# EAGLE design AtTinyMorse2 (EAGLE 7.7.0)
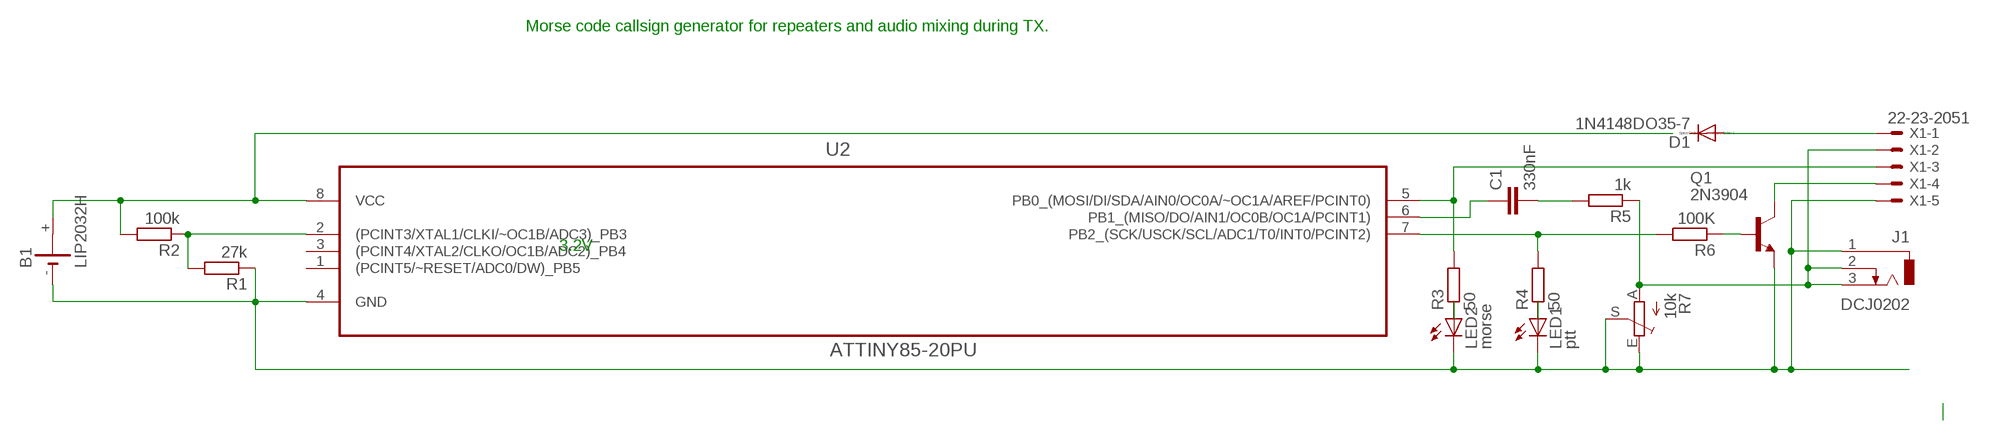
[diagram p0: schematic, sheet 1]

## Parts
B1  LIP2032H  CR2032H  [CR2032H]
C1  330nF  C5/2.5  [C5B2.5]
D1  1N4148DO35-7  [DO35-7]
J1  DCJ0202  [DCJ0202]
LED1  ptt  LED3MM  [LED3MM]
LED2  morse  LED3MM  [LED3MM]
Q1  2N3904  [TO92]
R1  27k  R-EU_0204/7  [0204/7]
R2  100k  R-EU_0204/7  [0204/7]
R3  50  R-EU_0204/7  [0204/7]
R4  50  R-EU_0204/7  [0204/7]
R5  1k  R-EU_0204/7  [0204/7]
R6  100K  R-EU_0204/7  [0204/7]
R7  10k  TRIM_EU-LI10  [LI10]
U2  ATTINY85-20PU  [DIP254P762X533-8]
X1  22-23-2051  [22-23-2051]

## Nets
N$1: LED2.A R3.1
N$2: LED1.A R4.1
N$4: Q1.1(C) X1.4
N$9: C1.2 R5.2
N$10: J1.2 J1.3 R5.1 R7.A X1.2
N$12: Q1.2(B) R6.1
N$13: D1.A X1.1
N$14: B1.- J1.1 LED1.K(C) LED2.K(C) R1.1 R7.E R7.S U2.4(GND) X1.5
N$15: B1.+ R2.2 U2.8(VCC)
N$16: R1.2 R2.1 U2.2((PCINT3/XTAL1/CLKI/~OC1B/ADC3)_PB3)
N$19: Q1.3(E)
N$20: R4.2 R6.2 U2.7(PB2_(SCK/USCK/SCL/ADC1/T0/INT0/PCINT2))
N$21: R3.2 U2.5(PB0_(MOSI/DI/SDA/AIN0/OC0A/~OC1A/AREF/PCINT0)) X1.3
N$22: C1.1 U2.6(PB1_(MISO/DO/AIN1/OC0B/OC1A/PCINT1))
Unconnected: B1.+@1(+) D1.C U2.1((PCINT5/~RESET/ADC0/DW)_PB5) U2.3((PCINT4/XTAL2/CLKO/OC1B/ADC2)_PB4)

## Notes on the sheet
- Morse code callsign generator for repeaters and audio mixing during TX.
- 3.2V

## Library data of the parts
B1 = battery:CR2032H: LI BATTERY Varta
C1 = capacitor-wima:C: CAPACITOR
D1 = diode:1N4148: DIODE
J1 = con-jack:DCJ0202: DC POWER JACK Source: DCJ0202.pdf; OC_FARNELL: unknown; OC_NEWARK: unknown
LED1 LED2 = led:LED: LED
Q1 = transistor-npn:2N3904: NPN Transistor
R1-R6 = resistor:R-EU_: RESISTOR, European symbol
R7 = pot:TRIM_EU-: POTENTIOMETER
U2 = Atmel_By_element14_Batch_1-00:ATTINY85-20PU: 8-bit Microcontroller with In-System Programmable Flash; MPN: ATTINY85-20PU; OC_FARNELL: 1455162; OC_NEWARK: 58M3796; PACKAGE: PDIP-8; SUPPLIER: Atmel
X1 = con-molex:22-23-2051: .100" (2.54mm) Center Header - 5 Pin; MF: MOLEX; MPN: 22-23-2051; OC_FARNELL: 1462952; OC_NEWARK: 38C9178

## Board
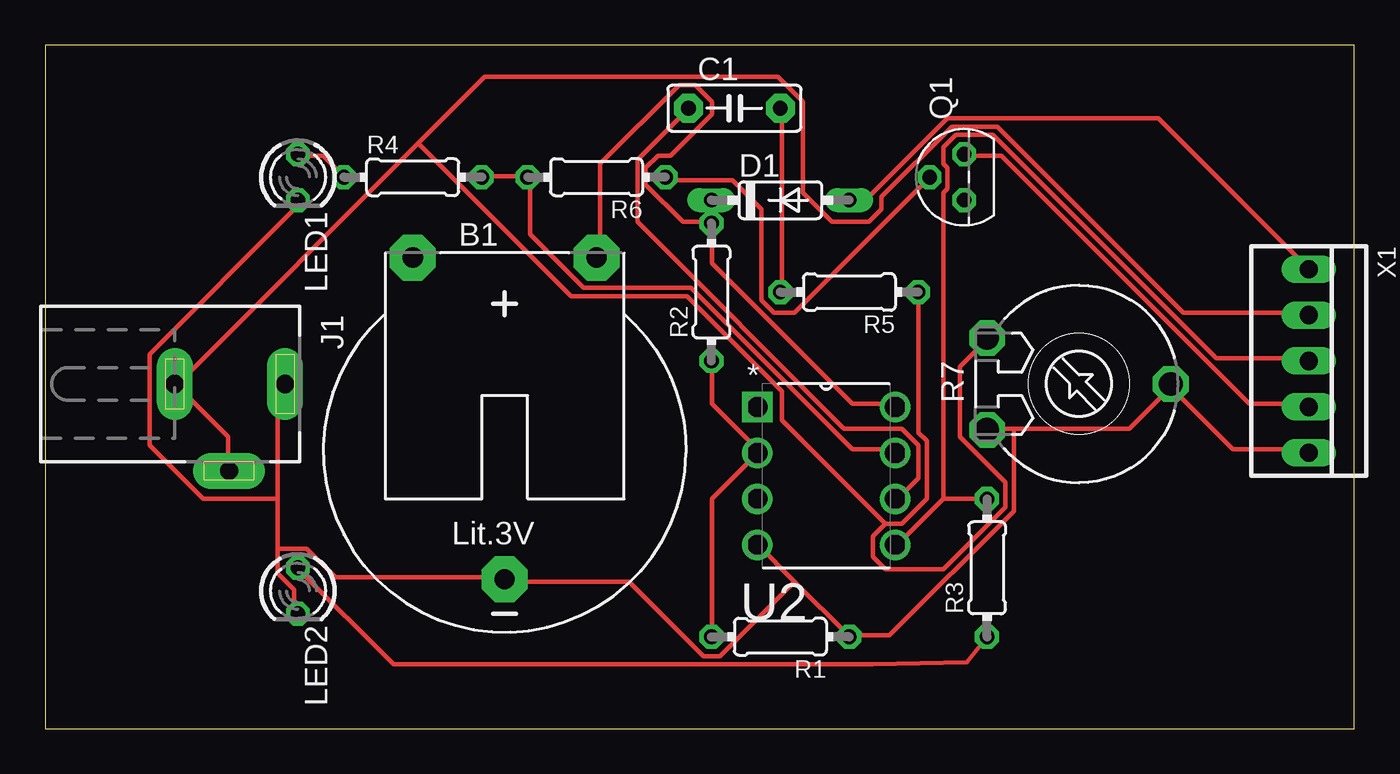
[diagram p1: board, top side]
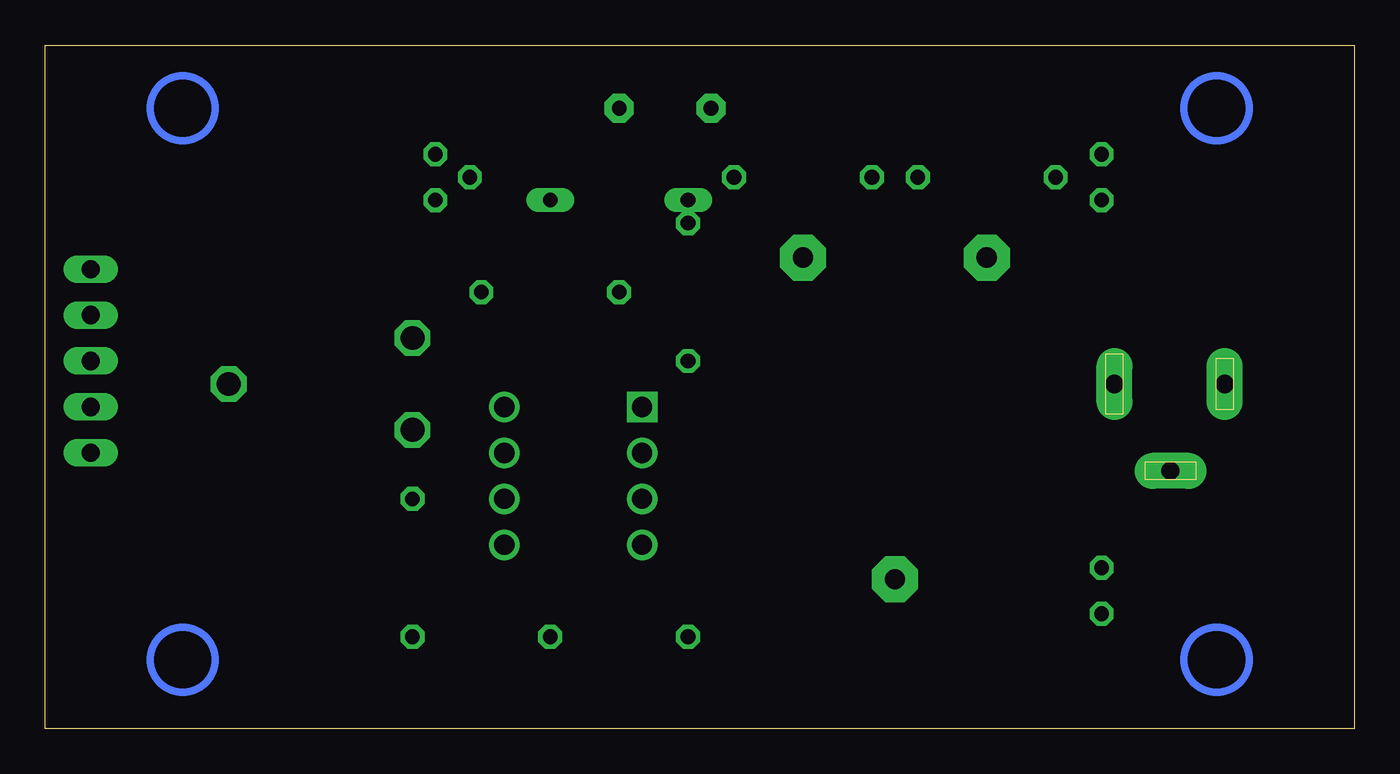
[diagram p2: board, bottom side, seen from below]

Size 72.37 x 37.77 mm. Coordinates in mm from the lower left corner, seen from the top.
Outline: 0,0 72.37,0 72.37,37.77 0,37.77 0,0
Copper layers (1*16): Top 0.035mm / dielectric 1.5mm / Bottom 0.035mm
Design rules "default": minimum track width 10mil, minimum drill 24mil, track to track 8mil, track to pad 8mil, pad to pad 8mil, via to via 8mil, smd to smd 8mil, copper to edge 40mil, drill to drill 8mil, minimum pad ring 10mil, minimum via ring 8mil, stop-mask expansion 4mil, vias tented up to drill 0mil, thermal gap 10mil

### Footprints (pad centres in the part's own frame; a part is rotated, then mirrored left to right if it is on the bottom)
CR2032H = drill 1.118 pad 2.54 octagon: + 5.08,10.795; +@1 -5.08,10.795; - 0,-6.985
C5B2.5 = drill 0.813 pad 1.6 octagon: 1 -2.54,0; 2 2.54,0
DO35-7 = drill 0.813 long: A 3.81,0; C -3.81,0
DCJ0202 = drill 1 pad 2 long: 1 0,3.1; 2 4.8,0; 3 0,-3
LED3MM = drill 0.813 octagon: A -1.27,0; K 1.27,0
TO92 = drill 0.813 octagon: 1 1.27,0; 2 0,1.905; 3 -1.27,0
0204/7 = drill 0.813 octagon: 1 -3.81,0; 2 3.81,0
LI10 = drill 1.321 octagon: A -2.54,-5.08; E 2.54,-5.08; S 0,5.08
DIP254P762X533-8 = drill 1.118 square: 1 -7.62,7.62 | drill 1.118: 2 -7.62,5.08; 3 -7.62,2.54; 4 -7.62,0; 5 0,0; 6 0,2.54; 7 0,5.08; 8 0,7.62
22-23-2051 = drill 1 long: 1 -5.08,0; 2 -2.54,0; 3 0,0; 4 2.54,0; 5 5.08,0

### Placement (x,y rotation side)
B1  25.4,15.24 0 top
C1  38.1,34.29 0 top
D1  40.64,29.21 0 top
J1  10.16,19.05 270 top
LED1  13.97,30.48 270 top
LED2  13.97,7.62 270 top
Q1  50.8,30.48 90 top
R1  40.64,5.08 180 top
R2  36.83,24.13 90 top
R3  52.07,8.89 90 top
R4  20.32,30.48 0 top
R5  44.45,24.13 180 top
R6  30.48,30.48 180 top
R7  57.15,19.05 270 top
U2  46.99,10.16 0 top
X1  69.85,20.32 270 top

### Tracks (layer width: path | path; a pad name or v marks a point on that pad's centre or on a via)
N$1
  Top 0.254: R3.1 51.94,4.93 50.95,3.66 45.77,3.56 19.25,3.56 13.99,8.81 LED2.A
N$2
  Top 0.254: LED1.A 13.99,31.67 15.37,31.67 16.51,30.53 R4.1
N$4
  Top 0.254: Q1.1 50.8,31.67 52.86,31.67 66.57,17.96 69.77,17.96 X1.4
N$9
  Top 0.254: R5.2 40.74,24.13 40.74,34.19 C1.2
N$10
  Top 0.254: 46.46,11.33 47.37,11.33 48.74,12.7 48.74,15.9 48.28,16.36 48.28,24.13 R5.1 | 46.46,11.33 45.77,10.64 45.77,9.5 46.46,8.81 49.66,8.81 53.09,12.24 53.09,13.61 50.57,16.13 50.57,20.02 51.94,21.39 R7.A | 20.62,32.36 7.37,19.1 J1.3 7.37,18.87 10.11,16.13 10.11,14.3 J1.2 | 20.62,32.36 24.28,36.02 40.51,36.02 41.88,34.65 41.88,29.62 43.48,28.02 45.54,28.02 46.23,28.7 46.23,29.39 50.11,33.27 52.63,33.27 62.92,22.99 69.77,22.99 X1.2 | 46.46,11.33 40.74,17.04 40.74,18.64 35.48,23.9 29.08,23.9 20.62,32.36
N$12
  Top 0.254: R6.1 34.34,30.3 38,30.3 39.6,28.7 39.6,23.67 40.28,22.99 41.43,22.99 48.74,30.3 Q1.2
N$13
  Top 0.254: D1.A 44.63,29.39 45.54,29.39 49.89,33.73 61.54,33.73 69.77,25.5 X1.1
N$14
  Top 0.254: 12.85,12.7 12.85,18.64 13.08,18.87 J1.1 | 12.85,12.7 12.85,9.96 | 12.85,9.96 12.85,8.59 13.77,7.67 13.77,6.53 LED2.K | 12.85,12.7 8.74,12.7 5.77,15.67 5.77,20.7 13.77,28.7 13.77,29.16 LED1.K | 12.85,9.96 14.45,9.96 16.05,8.36 25.2,8.36 B1.- 25.42,8.13 32.28,8.13 36.4,4.01 37.31,4.01 41.43,8.13 | 41.43,8.13 39.37,10.18 U2.4 | 41.43,8.13 44.4,5.16 R1.1 44.63,5.16 46.68,5.16 53.54,12.01 53.54,16.59 | 62.23,18.87 65.66,15.44 69.77,15.44 X1.5 | 53.54,16.59 59.94,16.59 62.23,18.87 | 53.54,16.59 52.17,16.59 R7.E | 62.23,18.87 R7.S
N$15
  Top 0.254: U2.8 46.91,17.96 44.63,17.96 36.85,25.73 36.85,27.79 R2.2 36.63,28.02 35.26,28.02 33.2,30.07 33.2,30.99 33.88,31.67 34.57,31.67 36.85,33.96 36.85,34.65 35.94,35.56 35.03,35.56 30.68,31.22 30.68,26.19 B1.+
N$16
  Top 0.254: R1.2 36.85,5.16 36.85,12.7 39.37,15.21 U2.2 39.37,15.44 36.85,17.96 36.85,20.24 R2.1
N$20
  Top 0.254: R4.2 24.28,30.53 26.57,30.53 R6.2 26.8,30.3 26.8,27.33 29.77,24.36 35.71,24.36 44.63,15.44 46.91,15.44 U2.7
N$21
  Top 0.254: 49.66,12.7 R3.2 | 49.66,12.7 47.14,10.18 U2.5 | 49.66,12.7 49.66,29.62 49.89,29.84 49.89,30.99 49.66,31.22 49.66,32.13 50.34,32.82 52.4,32.82 64.75,20.47 69.77,20.47 X1.3
N$22
  Top 0.254: C1.1 35.48,34.19 32.74,31.45 32.74,28.02 44.17,16.59 47.37,16.59 48.28,15.67 48.28,13.84 47.14,12.7 U2.6
(copper drawn outside any net)
  shapes: Bottom circle x4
